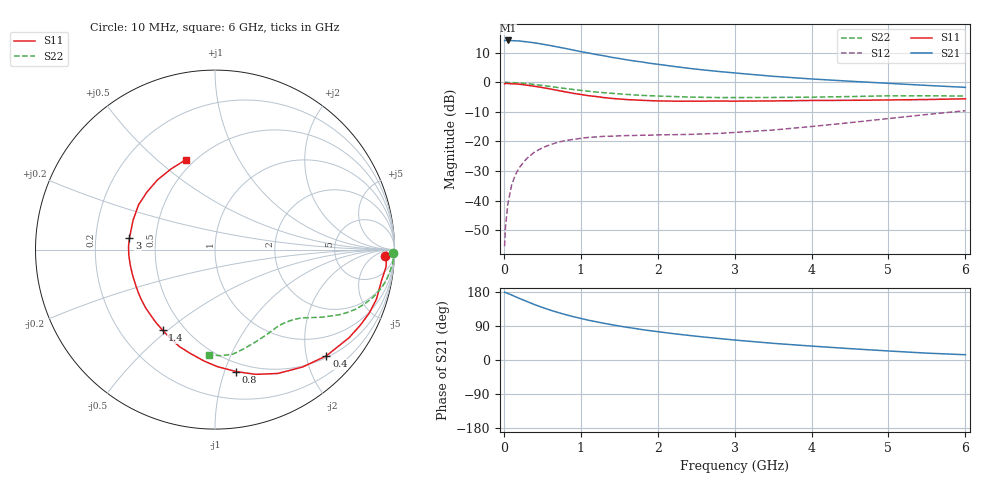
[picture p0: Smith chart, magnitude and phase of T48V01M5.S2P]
! Infineon Technologies  Discrete & RF Semiconductors
! BFR182T
! Si NPN RF Bipolar Junction Transistor in SC75
! VCE = 8 V  IC = 1.5 mA
! Common Emitter S-Parameters:  October  1999
# GHz  S  MA  R  50
!  f  S11  S21  S12  S22
! GHz  MAG  ANG  MAG  ANG  MAG  ANG  MAG  ANG
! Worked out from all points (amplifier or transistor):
!   36 points, 10 MHz to 6 GHz, reference 50 ohm
!   highest |S21| = 14.2 dB at 50 MHz (marker M1)
!   |S21| within 3 dB of that: start of sweep to 856.5 MHz
!   unconditionally stable (mu >= 1): 2.238 GHz to 4.515 GHz
!   at 250 MHz: K = 0.11, MSG = 20.5 dB, |S12| = -27.2 dB
!   at 1.4 GHz: K = 0.67, MSG = 13.3 dB, |S12| = -18.2 dB
!   at 6 GHz: K = 0.83, MSG = 3.9 dB, |S12| = -9.6 dB
!   S11 on the Smith chart (normalised r, x): 10 MHz: 24, -17; 400 MHz: 0.54, -2.40; 800 MHz: 0.42, -1.10; 1.4 GHz: 0.38, -0.48; 3 GHz: 0.35, +0.06; 6 GHz: 0.45, +0.62
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0.01  0.9453 -2.2  5.08 178.4  0.0017 89.7  0.9898 -1.2
0.02  0.9572 -0.8  5.097 178.6  0.0034 94.8  0.999 -1.0
0.05  0.9576 -5.8  5.103 175.7  0.0085 89.7  0.9947 -2.4
0.1  0.9431 -10.9  5.067 171.7  0.0181 84.9  0.9931 -4.6
0.15  0.941 -17.1  5.041 167.1  0.0275 79.4  0.9825 -6.9
0.25  0.9126 -27.5  4.912 158.6  0.0436 74.4  0.9635 -11.1
0.4  0.8577 -43.6  4.653 146.1  0.0664 65.6  0.919 -16.9
0.5  0.816 -53.3  4.422 138.9  0.078 60.8  0.8863 -20.0
0.6  0.7738 -63.1  4.194 131.8  0.0881 56.3  0.8523 -22.9
0.8  0.69 -80.1  3.742 119.8  0.1037 49.3  0.7864 -27.4
0.9  0.6528 -88.7  3.516 114.5  0.1083 46.7  0.7565 -29.1
1.1  0.5951 -103.2  3.134 104.9  0.1172 42.4  0.7079 -32.1
1.4  0.5354 -123.1  2.65 93.2  0.1228 38.4  0.6526 -35.5
1.6  0.5107 -135.2  2.399 86.3  0.1259 37.3  0.6244 -37.5
1.8  0.4962 -145.8  2.2 80.1  0.1276 36.9  0.6016 -39.7
2.2  0.4809 -162.5  1.865 69.6  0.1304 38.2  0.5753 -43.6
2.6  0.4812 -176.3  1.617 60.6  0.1345 41.6  0.5575 -48.3
3  0.481 172.4  1.441 52.7  0.1421 45.6  0.5522 -52.7
3.5  0.485 160.2  1.265 44.0  0.1563 51.1  0.555 -59.4
4.5  0.4965 139.9  1.044 30.0  0.2082 57.8  0.5748 -73.2
5.5  0.5119 118.5  0.887 18.1  0.2861 58.1  0.5925 -86.8
6  0.5264 108.1  0.822 13.9  0.3315 55.6  0.5861 -93.1
